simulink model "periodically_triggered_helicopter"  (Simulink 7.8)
settings: Solver=ode45  StartTime=0.0  StopTime=89  RelTol=1e-3
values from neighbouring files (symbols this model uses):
  d = lambda*0.5    [main_epsilon.m]    (also in main_rho_tau.m = 0.5)
undefined symbols (not defined in the file or in its folder): Ac_epsilon, Ac_rho, Ac_tau, c_epsilon, DiscIntNeverNeededParam, epsilon_0, Epsilon_disc, g, J_epsilon, Ka, Kb, Kc, L_epsilon, L_rho, L_tau, la, lh, lw, m, M, M_bf, Rho_disc, Tau_disc
libraries: simulink x6, commnoisgen2 x6, dspswit3 x3

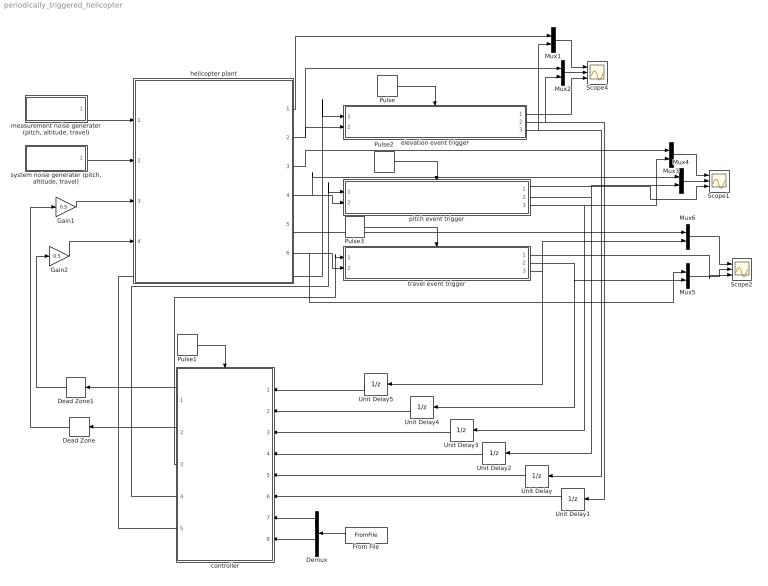
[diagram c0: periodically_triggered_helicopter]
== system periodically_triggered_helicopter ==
  Dead Zone : DeadZone  LowerValue=-1  UpperValue=1
  Dead Zone1 : DeadZone  LowerValue=-1  UpperValue=1
  Demux : Demux  Outputs=2
  From File : FromFile  FileName=input.mat  SampleTime=0
  Gain1 : Gain  Gain=0.5
  Gain2 : Gain  Gain=0.5
  Mux{1..6} (6 alike) : Mux  Inputs=2
  Pulse : DiscretePulseGenerator  PulseType=Time based  Period=0.005  PulseWidth=50
  Pulse1 : DiscretePulseGenerator  PulseType=Time based  Period=0.005  PulseWidth=30
  Pulse2 : DiscretePulseGenerator  PulseType=Time based  Period=0.005  PulseWidth=50
  Pulse3 : DiscretePulseGenerator  PulseType=Time based  Period=0.005  PulseWidth=50
  Scope1 : Scope  NumInputPorts=3
  Scope2 : Scope  NumInputPorts=3
  Scope4 : Scope  NumInputPorts=3
  Unit Delay{,1..5} (6 alike) : UnitDelay  SampleTime=-1
  controller : Subsystem
  elevation event trigger : Subsystem
  helicopter plant : Subsystem
  "measurement noise generater (pitch, altitude, travel)" : Subsystem
  pitch event trigger : Subsystem
  "system noise generater (pitch, altitude, travel)" : Subsystem
  travel event trigger : Subsystem
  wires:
  helicopter plant/2(altitude) -> elevation event trigger/2(elevation), Mux2/1
  Pulse/1 -> elevation event trigger/Trigger
  Mux1/1 -> Scope4/1
  Pulse1/1 -> controller/Trigger
  helicopter plant/5(travel rate) -> Mux6/1
  helicopter plant/3(pitch rate) -> Mux3/1
  controller/1(Vb) -> Dead Zone1/1
  Gain2/1 -> helicopter plant/4(Tb)
  controller/2(Vf) -> Dead Zone/1
  Gain1/1 -> helicopter plant/3(Tf)
  controller/5(u_elv) -> elevation event trigger/1(u_elv)
  From File/1 -> Demux/1
  Demux/2 -> controller/8(travel_rate_offset)
  Demux/1 -> controller/7(elevation_offset)
  helicopter plant/1(altitude rate) -> Mux1/1
  Mux2/1 -> Scope4/2
  elevation event trigger/3(remote estimated elevation rate) -> Unit Delay/1, Mux1/2
  elevation event trigger/2(remote estimated elevation) -> Unit Delay1/1, Mux2/2
  elevation event trigger/1(elevation transmission times) -> Scope4/3
  Pulse2/1 -> pitch event trigger/Trigger
  Unit Delay/1 -> controller/5(elevation_rate)
  Unit Delay1/1 -> controller/6(elevation)
  helicopter plant/4(pitch) -> pitch event trigger/2(pitch), Mux4/1
  pitch event trigger/2(remote estimated pitch) -> Unit Delay2/1, Mux4/2
  Unit Delay2/1 -> controller/4(pitch)
  pitch event trigger/3(remote estimated pitch rate) -> Mux3/2, Unit Delay3/1
  Mux3/1 -> Scope1/1
  Mux4/1 -> Scope1/2
  pitch event trigger/1(pitch transmission interval) -> Scope1/3
  Pulse3/1 -> travel event trigger/Trigger
  helicopter plant/6(travel) -> travel event trigger/2(travel), Mux5/1
  controller/3(u_trv) -> travel event trigger/1(u_trv)
  controller/4(u_pth) -> pitch event trigger/1(u_pth)
  Mux5/1 -> Scope2/2
  travel event trigger/2("remote estimated travel ") -> Unit Delay4/1, Mux5/2
  Unit Delay3/1 -> controller/3(pitch_rate)
  Unit Delay4/1 -> controller/2(travel)
  travel event trigger/3(remote estimated travel rate) -> Mux6/2, Unit Delay5/1
  Mux6/1 -> Scope2/1
  travel event trigger/1(travel transmission interval) -> Scope2/3
  Unit Delay5/1 -> controller/1(travel_rate)
  "measurement noise generater (pitch, altitude, travel)"/1(measurement noise) -> helicopter plant/1("measurement noise (pitch, altitude, travel)")
  "system noise generater (pitch, altitude, travel)"/1(system noise) -> helicopter plant/2("system noise (pitch, altitude, travel)")
  Dead Zone/1 -> Gain1/1
  Dead Zone1/1 -> Gain2/1

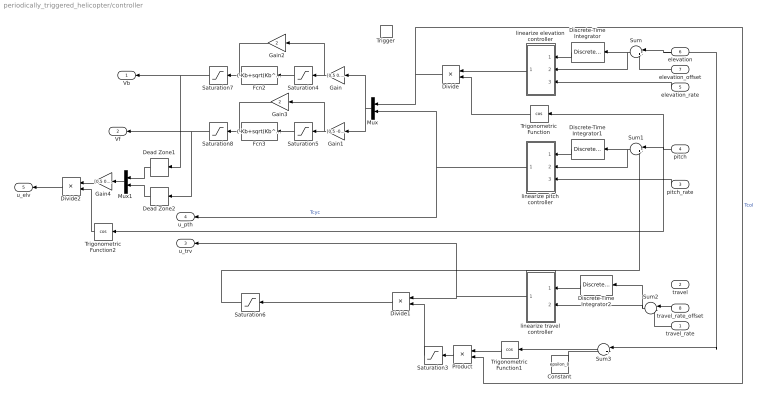
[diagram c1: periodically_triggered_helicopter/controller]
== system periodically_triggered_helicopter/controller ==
  travel_rate : Inport
  travel : Inport  Port=2
  pitch_rate : Inport  Port=3
  pitch : Inport  Port=4
  elevation_rate : Inport  Port=5
  elevation : Inport  Port=6
  elevation_offset : Inport  Port=7
  travel_rate_offset : Inport  Port=8
  Trigger : TriggerPort
  Constant : Constant  Value=epsilon_0
  Dead Zone1 : DeadZone  LowerValue=-1  UpperValue=1
  Dead Zone2 : DeadZone  LowerValue=-1  UpperValue=1
  Discrete-Time Integrator : DiscreteIntegrator  SampleTime=-1  LimitOutput=on  UpperSaturationLimit=1.8  LowerSaturationLimit=-1.8  ICPrevOutput=DiscIntNeverNeededParam  ICPrevScaledInput=DiscIntNeverNeededParam
  Discrete-Time Integrator1 : DiscreteIntegrator  SampleTime=-1  LimitOutput=on  UpperSaturationLimit=0.5  LowerSaturationLimit=-0.5  ICPrevOutput=DiscIntNeverNeededParam  ICPrevScaledInput=DiscIntNeverNeededParam
  Discrete-Time Integrator2 : DiscreteIntegrator  SampleTime=-1  LimitOutput=on  UpperSaturationLimit=0.12  LowerSaturationLimit=-0.12  ICPrevOutput=DiscIntNeverNeededParam  ICPrevScaledInput=DiscIntNeverNeededParam
  Divide : Product  Inputs=*/
  Divide1 : Product  Inputs=*/
  Divide2 : Product  Inputs=**
  Fcn2 : Fcn  Expr=(-Kb+sqrt(Kb^2-4*Ka*(Kc-u(1))))/(2*Ka)
  Fcn3 : Fcn  Expr=(-Kb+sqrt(Kb^2-4*Ka*(Kc-u(1))))/(2*Ka)
  Gain : Gain  Gain=[0.5 0.5]  Multiplication=Matrix(K*u)
  Gain1 : Gain  Gain=[0.5 -0.5]  Multiplication=Matrix(K*u)
  Gain2 : Gain  Gain=2
  Gain3 : Gain  Gain=2
  Gain4 : Gain  Gain=[0.5 0.5]  Multiplication=Matrix(K*u)
  Mux : Mux  Inputs=2
  Mux1 : Mux  Inputs=2
  Product : Product
  Saturation3 : Saturate  UpperLimit=inf  LowerLimit=0.8
  Saturation4 : Saturate  UpperLimit=1  LowerLimit=-0.0012
  Saturation5 : Saturate  UpperLimit=1  LowerLimit=-0.0012
  Saturation6 : Saturate  UpperLimit=0.6  LowerLimit=-0.6
  Saturation7 : Saturate  UpperLimit=4.99  LowerLimit=-4.99
  Saturation8 : Saturate  UpperLimit=4.99  LowerLimit=-4.99
  Sum : Sum  Inputs=|+-
  Sum1 : Sum  Inputs=|+-
  Sum2 : Sum  Inputs=|-+
  Sum3 : Sum  Inputs=|+-
  Trigonometric Function : Trigonometry  Operator=cos
  Trigonometric Function1 : Trigonometry  Operator=cos
  Trigonometric Function2 : Trigonometry  Operator=cos
  linearize elevation controller : Subsystem
  linearize pitch controller : Subsystem
  linearize travel controller : Subsystem
  Vb : Outport
  Vf : Outport  Port=2
  u_trv : Outport  Port=3
  u_pth : Outport  Port=4
  u_elv : Outport  Port=5
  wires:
  elevation/1 -> Sum/1, Sum3/1
  elevation_offset/1 -> Sum/2
  Sum/1 -> linearize elevation controller/2(P), Discrete-Time Integrator/1
  Discrete-Time Integrator/1 -> linearize elevation controller/1(I)
  elevation_rate/1 -> linearize elevation controller/3(D)
  pitch/1 -> Sum1/1, Trigonometric Function/1, Trigonometric Function2/1
  Sum1/1 -> linearize pitch controller/2(P), Discrete-Time Integrator1/1
  pitch_rate/1 -> linearize pitch controller/3(D)
  travel_rate_offset/1 -> Sum2/1
  travel_rate/1 -> Sum2/2
  Sum2/1 -> Discrete-Time Integrator2/1, linearize travel controller/2(P)
  Discrete-Time Integrator2/1 -> linearize travel controller/1(I)
  Sum3/1 -> Trigonometric Function1/1
  Trigonometric Function1/1 -> Product/1
  Divide/1 -> Mux/1, Product/2  "Tcol"
  Product/1 -> Saturation3/1
  Saturation3/1 -> Divide1/2
  Mux/1 -> Gain/1, Gain1/1
  Gain/1 -> Saturation4/1, Gain2/1
  Gain1/1 -> Saturation5/1, Gain3/1
  Divide1/1 -> Saturation6/1
  Saturation6/1 -> Sum1/2
  Saturation7/1 -> Vb/1, Dead Zone1/1
  Saturation8/1 -> Vf/1, Dead Zone2/1
  Constant/1 -> Sum3/2
  Saturation4/1 -> Fcn2/1
  Saturation5/1 -> Fcn3/1
  Trigonometric Function/1 -> Divide/2
  Discrete-Time Integrator1/1 -> linearize pitch controller/1(I)
  Gain2/1 -> Saturation7/1
  Gain3/1 -> Saturation8/1
  linearize pitch controller/1(u_pth) -> Mux/2, u_pth/1  "Tcyc"
  linearize travel controller/1(u_trv) -> Divide1/1, u_trv/1
  linearize elevation controller/1(u_elv) -> Divide/1
  Dead Zone1/1 -> Mux1/1
  Dead Zone2/1 -> Mux1/2
  Mux1/1 -> Gain4/1
  Gain4/1 -> Divide2/1
  Trigonometric Function2/1 -> Divide2/2
  Divide2/1 -> u_elv/1

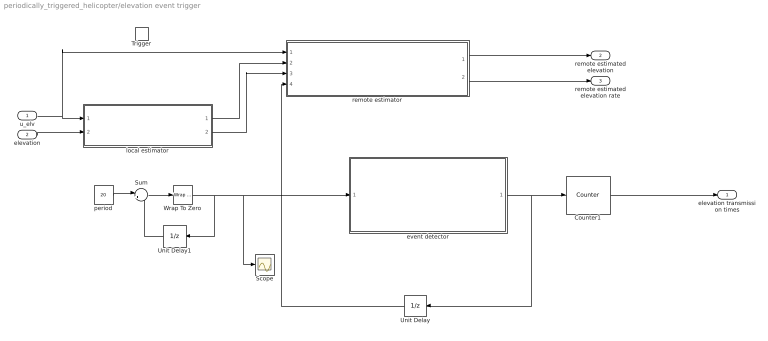
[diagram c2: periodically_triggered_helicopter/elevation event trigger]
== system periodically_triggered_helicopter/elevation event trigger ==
  u_elv : Inport
  elevation : Inport  Port=2
  Trigger : TriggerPort
  Counter1 : dspswit3/Counter  Direction=Up  CountEvent=Non-zero sample  CounterSize=User defined  MaxCount=20000  InitialCount=0  Output=Count  HitValue=32  ResetInput=off  SamplesPerFrame=1  Ts=1  CntDtype=int32  HitDtype=Logical
  Scope : Scope
  Sum : Sum  Inputs=|++
  Unit Delay : UnitDelay  SampleTime=-1
  Unit Delay1 : UnitDelay  SampleTime=-1
  Wrap To Zero : simulink/Discontinuities/Wrap To Zero  Threshold=4
  event detector : Subsystem
  local estimator : Subsystem
  period : Constant  Value=20
  remote estimator : Subsystem
  elevation transmission times : Outport
  remote estimated elevation : Outport  Port=2
  remote estimated elevation rate : Outport  Port=3
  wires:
  u_elv/1 -> local estimator/1(u_elv), remote estimator/1(u_elv)
  elevation/1 -> local estimator/2(elevation)
  local estimator/1(local estimated elevation) -> remote estimator/2("local estimated elevation ")
  remote estimator/1(remote estimated elevation) -> remote estimated elevation/1
  local estimator/2(local estimated elevation rate) -> remote estimator/3(local estimated elevation rate)
  event detector/1(transmit signal) -> Unit Delay/1, Counter1/1
  Counter1/1 -> elevation transmission times/1
  Unit Delay/1 -> remote estimator/4(transmit signal)
  remote estimator/2(remote estimated elevation rate) -> remote estimated elevation rate/1
  period/1 -> Sum/1
  Sum/1 -> Wrap To Zero/1
  Wrap To Zero/1 -> event detector/1(steps), Scope/1, Unit Delay1/1
  Unit Delay1/1 -> Sum/2

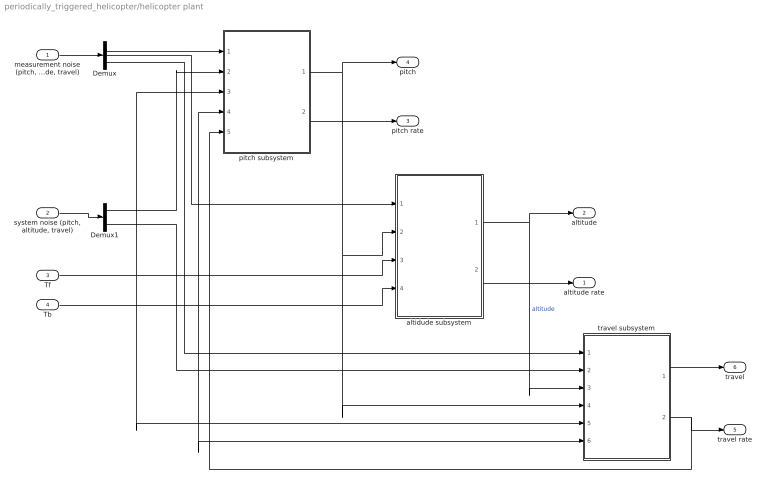
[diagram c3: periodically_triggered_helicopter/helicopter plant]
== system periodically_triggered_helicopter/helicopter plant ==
  "measurement noise (pitch, altitude, travel)" : Inport
  "system noise (pitch, altitude, travel)" : Inport  Port=2
  Tf : Inport  Port=3
  Tb : Inport  Port=4
  Demux : Demux  Outputs=3
  Demux1 : Demux  Outputs=3
  altidude subsystem : Subsystem
  pitch subsystem : Subsystem
  travel subsystem : Subsystem
  altitude rate : Outport
  altitude : Outport  Port=2
  pitch rate : Outport  Port=3
  pitch : Outport  Port=4
  travel rate : Outport  Port=5
  travel : Outport  Port=6
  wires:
  pitch subsystem/1(pitch) -> pitch/1, altidude subsystem/2(pitch), travel subsystem/4(pitch)
  altidude subsystem/1(altitude) -> altitude/1, travel subsystem/3(altitude)  "altitude"
  pitch subsystem/2(pitch rate) -> pitch rate/1
  altidude subsystem/2(altitude rate) -> altitude rate/1
  travel subsystem/1(travel) -> travel/1
  travel subsystem/2(travel rate) -> pitch subsystem/5(travel_rate), travel rate/1
  Demux/1 -> pitch subsystem/1(measurement noise)
  Demux/2 -> altidude subsystem/1(measurement noise)
  Demux/3 -> travel subsystem/1(measurement noise)
  "measurement noise (pitch, altitude, travel)"/1 -> Demux/1
  Demux1/1 -> pitch subsystem/2(system noise)
  Demux1/3 -> travel subsystem/2(system noise)
  Tf/1 -> altidude subsystem/3(Tf), travel subsystem/5(Tf), pitch subsystem/3(Tf)
  Tb/1 -> altidude subsystem/4(Tb), pitch subsystem/4(Tb), travel subsystem/6(Tb)
  "system noise (pitch, altitude, travel)"/1 -> Demux1/1

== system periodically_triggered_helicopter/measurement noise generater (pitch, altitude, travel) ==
  Mux : Mux  Inputs=3
  altitude Noise Generator : commnoisgen2/Gaussian Noise Generator  m=0  d=1.857e-8  s=41  Ts=0.0025  frameBased=off  sampPerFrame=1  orient=off  outDataType=double
  pitch noise Generator : commnoisgen2/Gaussian Noise Generator  m=0  d=1.857e-8  s=1  Ts=0.0025  frameBased=off  sampPerFrame=1  orient=off  outDataType=double
  travel noise Generator : commnoisgen2/Gaussian Noise Generator  m=0  d=1.857e-8  s=3  Ts=0.0025  frameBased=off  sampPerFrame=1  orient=off  outDataType=double
  measurement noise : Outport
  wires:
  pitch noise Generator/1 -> Mux/1
  altitude Noise Generator/1 -> Mux/2
  travel noise Generator/1 -> Mux/3
  Mux/1 -> measurement noise/1

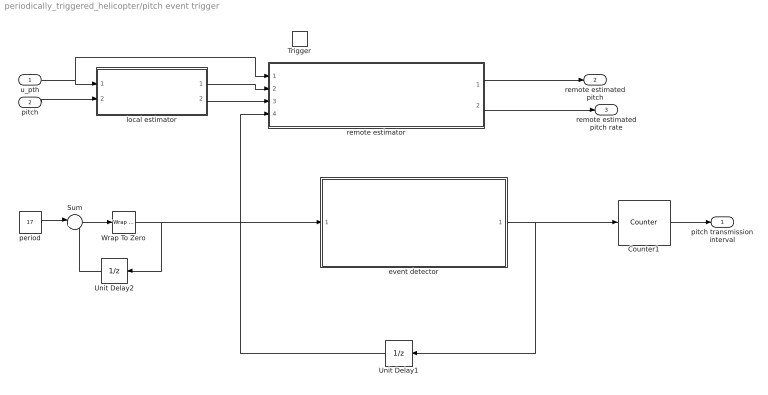
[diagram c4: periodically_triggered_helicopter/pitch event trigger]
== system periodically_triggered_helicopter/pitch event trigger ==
  u_pth : Inport
  pitch : Inport  Port=2
  Trigger : TriggerPort
  Counter1 : dspswit3/Counter  Direction=Up  CountEvent=Non-zero sample  CounterSize=User defined  MaxCount=20000  InitialCount=0  Output=Count  HitValue=32  ResetInput=off  SamplesPerFrame=1  Ts=1  CntDtype=int32  HitDtype=Logical
  Sum : Sum  Inputs=|++
  Unit Delay1 : UnitDelay  SampleTime=-1
  Unit Delay2 : UnitDelay  SampleTime=-1
  Wrap To Zero : simulink/Discontinuities/Wrap To Zero  Threshold=1
  event detector : Subsystem
  local estimator : Subsystem
  period : Constant  Value=17
  remote estimator : Subsystem
  pitch transmission interval : Outport
  remote estimated pitch : Outport  Port=2
  remote estimated pitch rate : Outport  Port=3
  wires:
  u_pth/1 -> local estimator/1(u_pth), remote estimator/1(u_pth)
  pitch/1 -> local estimator/2(pitch)
  local estimator/1(local estimated pitch) -> remote estimator/2(local estimated pitch)
  local estimator/2(local estimated pitch rate) -> remote estimator/3(local estimated pitch rate)
  remote estimator/1(remote estimated elevation) -> remote estimated pitch/1
  remote estimator/2(remote estimated elevation rate) -> remote estimated pitch rate/1
  Counter1/1 -> pitch transmission interval/1
  event detector/1(transmit signal) -> Unit Delay1/1, Counter1/1
  Unit Delay1/1 -> remote estimator/4(transmit signal)
  period/1 -> Sum/1
  Sum/1 -> Wrap To Zero/1
  Wrap To Zero/1 -> Unit Delay2/1, event detector/1(steps)
  Unit Delay2/1 -> Sum/2

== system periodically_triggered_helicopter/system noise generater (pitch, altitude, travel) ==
  Mux : Mux  Inputs=3
  altitude Noise Generator : commnoisgen2/Gaussian Noise Generator  m=0  d=1e-12  s=7  Ts=0.0025  frameBased=off  sampPerFrame=1  orient=off  outDataType=double
  pitch noise Generator : commnoisgen2/Gaussian Noise Generator  m=0  d=1e-12  s=5  Ts=0.0025  frameBased=off  sampPerFrame=1  orient=off  outDataType=double
  travel Noise Generator : commnoisgen2/Gaussian Noise Generator  m=0  d=1e-12  s=11  Ts=0.0025  frameBased=off  sampPerFrame=1  orient=off  outDataType=double
  system noise : Outport
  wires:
  pitch noise Generator/1 -> Mux/1
  altitude Noise Generator/1 -> Mux/2
  Mux/1 -> system noise/1
  travel Noise Generator/1 -> Mux/3

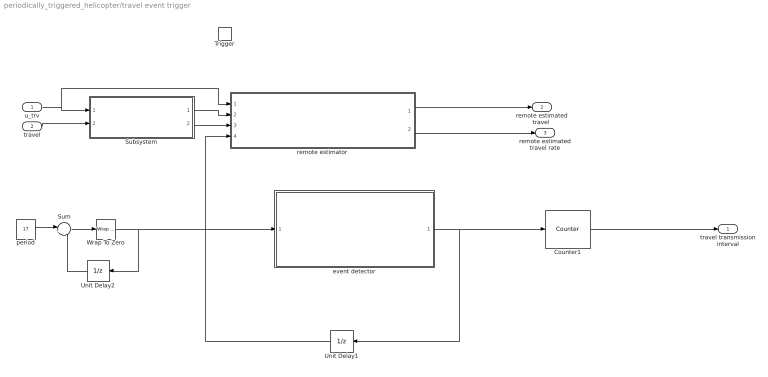
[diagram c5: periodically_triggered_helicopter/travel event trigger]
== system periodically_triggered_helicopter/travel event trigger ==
  u_trv : Inport
  travel : Inport  Port=2
  Trigger : TriggerPort
  Counter1 : dspswit3/Counter  Direction=Up  CountEvent=Non-zero sample  CounterSize=User defined  MaxCount=20000  InitialCount=0  Output=Count  HitValue=32  ResetInput=off  SamplesPerFrame=1  Ts=1  CntDtype=int32  HitDtype=Logical
  Subsystem : Subsystem
  Sum : Sum  Inputs=|++
  Unit Delay1 : UnitDelay  SampleTime=-1
  Unit Delay2 : UnitDelay  SampleTime=-1
  Wrap To Zero : simulink/Discontinuities/Wrap To Zero  Threshold=2
  event detector : Subsystem
  period : Constant  Value=17
  remote estimator : Subsystem
  travel transmission interval : Outport
  "remote estimated travel " : Outport  Port=2
  remote estimated travel rate : Outport  Port=3
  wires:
  u_trv/1 -> Subsystem/1(u_trv), remote estimator/1(u_trv)
  travel/1 -> Subsystem/2(travel)
  Subsystem/2(local estimated travel rate) -> remote estimator/3(local estimated travel rate)
  remote estimator/2(remote estimated travel rate) -> remote estimated travel rate/1
  remote estimator/1(remote estimated travel) -> "remote estimated travel "/1
  Subsystem/1(local estimated travel) -> remote estimator/2(local estimated travel)
  Counter1/1 -> travel transmission interval/1
  event detector/1(transmit signal) -> Unit Delay1/1, Counter1/1
  Unit Delay1/1 -> remote estimator/4(transmit signal)
  period/1 -> Sum/1
  Sum/1 -> Wrap To Zero/1
  Wrap To Zero/1 -> Unit Delay2/1, event detector/1(steps)
  Unit Delay2/1 -> Sum/2

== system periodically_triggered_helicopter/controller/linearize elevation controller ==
  I : Inport
  P : Inport  Port=2
  D : Inport  Port=3
  Gain : Gain  Gain=[-7 -44 -68]  Multiplication=Matrix(K*u)
  Mux : Mux  Inputs=3
  u_elv : Outport
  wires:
  Mux/1 -> Gain/1
  I/1 -> Mux/1
  Gain/1 -> u_elv/1
  P/1 -> Mux/2
  D/1 -> Mux/3

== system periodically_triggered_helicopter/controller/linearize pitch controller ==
  I : Inport
  P : Inport  Port=2
  D : Inport  Port=3
  Gain : Gain  Gain=[-3.5 -30 -20]  Multiplication=Matrix(K*u)
  Mux : Mux  Inputs=3
  u_pth : Outport
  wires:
  Mux/1 -> Gain/1
  I/1 -> Mux/1
  Gain/1 -> u_pth/1
  P/1 -> Mux/2
  D/1 -> Mux/3

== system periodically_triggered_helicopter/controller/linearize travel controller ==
  I : Inport
  P : Inport  Port=2
  Gain : Gain  Gain=[5 30]  Multiplication=Matrix(K*u)
  Mux : Mux  Inputs=2
  u_trv : Outport
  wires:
  Mux/1 -> Gain/1
  I/1 -> Mux/1
  Gain/1 -> u_trv/1
  P/1 -> Mux/2

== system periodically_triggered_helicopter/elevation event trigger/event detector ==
  steps : Inport
  Compare To Constant : simulink/Logic and Bit Operations/Compare To Constant  relop===  const=0  OutDataTypeStr=uint8
  transmit signal : Outport
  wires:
  steps/1 -> Compare To Constant/1
  Compare To Constant/1 -> transmit signal/1

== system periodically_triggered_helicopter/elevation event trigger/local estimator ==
  u_elv : Inport
  elevation : Inport  Port=2
  Demux : Demux  Outputs=2
  Gain2 : Gain  Gain=[Ac_epsilon(2:3,2:3) Epsilon_disc.B(2:3) L_epsilon(2:3,2)]  Multiplication=Matrix(K*u)
  Mux : Mux  Inputs=3
  Unit Delay : UnitDelay  SampleTime=-1
  local estimated elevation : Outport
  local estimated elevation rate : Outport  Port=2
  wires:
  Unit Delay/1 -> Mux/1
  u_elv/1 -> Mux/2
  elevation/1 -> Mux/3
  Mux/1 -> Gain2/1
  Gain2/1 -> Demux/1, Unit Delay/1
  Demux/1 -> local estimated elevation/1
  Demux/2 -> local estimated elevation rate/1

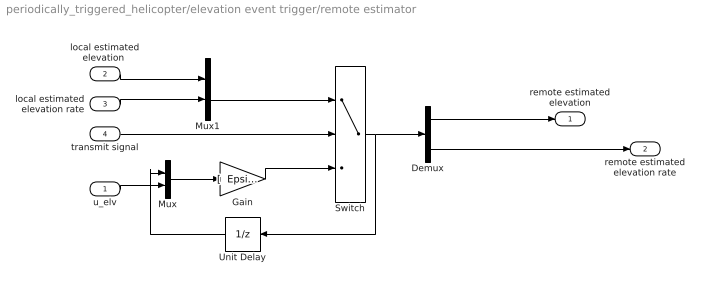
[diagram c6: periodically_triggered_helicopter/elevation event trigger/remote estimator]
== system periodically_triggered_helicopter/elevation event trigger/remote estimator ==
  u_elv : Inport
  "local estimated elevation " : Inport  Port=2
  local estimated elevation rate : Inport  Port=3
  transmit signal : Inport  Port=4
  Demux : Demux  Outputs=2
  Gain : Gain  Gain="[  Epsilon_disc.A(2:3,2:3)  Epsilon_disc.B(2:3)]"  Multiplication=Matrix(K*u)
  Mux : Mux  Inputs=2
  Mux1 : Mux  Inputs=2
  Switch : Switch  Threshold=1
  Unit Delay : UnitDelay  SampleTime=-1
  remote estimated elevation : Outport
  remote estimated elevation rate : Outport  Port=2
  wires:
  Mux/1 -> Gain/1
  u_elv/1 -> Mux/2
  Demux/1 -> remote estimated elevation/1
  Demux/2 -> remote estimated elevation rate/1
  Gain/1 -> Switch/3
  transmit signal/1 -> Switch/2
  Switch/1 -> Demux/1, Unit Delay/1
  Unit Delay/1 -> Mux/1
  "local estimated elevation "/1 -> Mux1/1
  local estimated elevation rate/1 -> Mux1/2
  Mux1/1 -> Switch/1

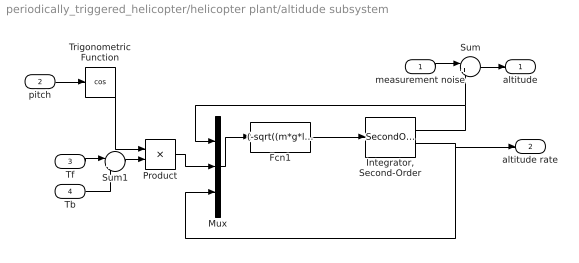
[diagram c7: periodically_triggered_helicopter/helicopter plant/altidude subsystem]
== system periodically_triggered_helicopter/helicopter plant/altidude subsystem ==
  measurement noise : Inport
  pitch : Inport  Port=2
  Tf : Inport  Port=3
  Tb : Inport  Port=4
  Fcn1 : Fcn  Expr=(-sqrt((m*g*lw-M*g*la)^2+((m+M)*g*d)^2)*sin(u(1))+(la+d*tan(u(1)+epsilon_0))*u(2)-c_epsilon*u(3))/J_epsilon
  "Integrator, Second-Order" : SecondOrderIntegrator
  Mux : Mux  Inputs=3
  Product : Product
  Sum : Sum  Inputs=|++
  Sum1 : Sum  Inputs=|++
  Trigonometric Function : Trigonometry  Operator=cos
  altitude : Outport
  altitude rate : Outport  Port=2
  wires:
  Fcn1/1 -> "Integrator, Second-Order"/1
  "Integrator, Second-Order"/1 -> Sum/2, Mux/1
  measurement noise/1 -> Sum/1
  Sum/1 -> altitude/1
  "Integrator, Second-Order"/2 -> altitude rate/1, Mux/3
  Tf/1 -> Sum1/1
  Tb/1 -> Sum1/2
  Mux/1 -> Fcn1/1
  Sum1/1 -> Product/2
  pitch/1 -> Trigonometric Function/1
  Product/1 -> Mux/2
  Trigonometric Function/1 -> Product/1

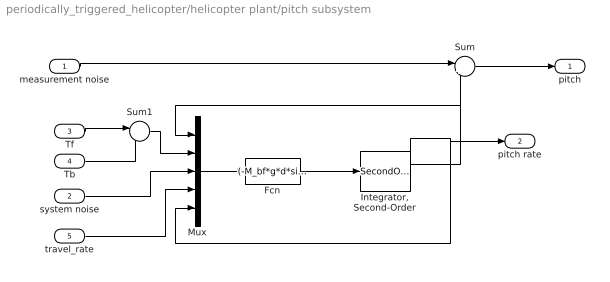
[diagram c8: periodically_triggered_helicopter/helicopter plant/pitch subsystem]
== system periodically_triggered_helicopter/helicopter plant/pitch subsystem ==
  measurement noise : Inport
  system noise : Inport  Port=2
  Tf : Inport  Port=3
  Tb : Inport  Port=4
  travel_rate : Inport  Port=5
  Fcn : Fcn  Expr=(-M_bf*g*d*sin(u(1))+lh*u(2)-0.003*u(5)+0.003*u(4)+u(3))/(0.01)
  "Integrator, Second-Order" : SecondOrderIntegrator
  Mux : Mux  Inputs=5
  Sum : Sum  Inputs=|++
  Sum1 : Sum  Inputs=|-+
  pitch : Outport
  pitch rate : Outport  Port=2
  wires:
  Mux/1 -> Fcn/1
  Fcn/1 -> "Integrator, Second-Order"/1
  "Integrator, Second-Order"/1 -> Sum/2, Mux/1
  measurement noise/1 -> Sum/1
  Sum/1 -> pitch/1
  "Integrator, Second-Order"/2 -> pitch rate/1, Mux/5
  system noise/1 -> Mux/3
  Tf/1 -> Sum1/1
  Tb/1 -> Sum1/2
  travel_rate/1 -> Mux/4
  Sum1/1 -> Mux/2

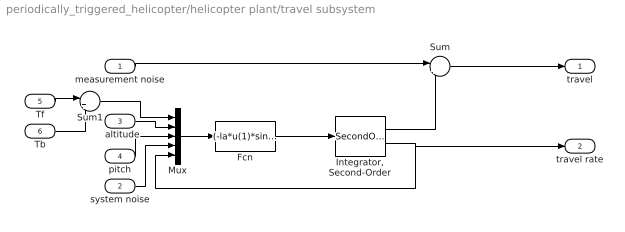
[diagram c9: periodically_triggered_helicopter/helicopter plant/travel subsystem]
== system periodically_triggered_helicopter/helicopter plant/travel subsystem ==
  measurement noise : Inport
  system noise : Inport  Port=2
  altitude : Inport  Port=3
  pitch : Inport  Port=4
  Tf : Inport  Port=5
  Tb : Inport  Port=6
  Fcn : Fcn  Expr=(-la*u(1)*sin(u(3))*cos(u(2)+epsilon_0)-0.25*u(5)+u(4))/4
  "Integrator, Second-Order" : SecondOrderIntegrator
  Mux : Mux  Inputs=5
  Sum : Sum  Inputs=|++
  Sum1 : Sum  Inputs=|++
  travel : Outport
  travel rate : Outport  Port=2
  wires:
  Mux/1 -> Fcn/1
  "Integrator, Second-Order"/1 -> Sum/2
  measurement noise/1 -> Sum/1
  Sum/1 -> travel/1
  altitude/1 -> Mux/2
  "Integrator, Second-Order"/2 -> travel rate/1, Mux/5
  Sum1/1 -> Mux/1
  pitch/1 -> Mux/3
  system noise/1 -> Mux/4
  Tf/1 -> Sum1/1
  Tb/1 -> Sum1/2
  Fcn/1 -> "Integrator, Second-Order"/1

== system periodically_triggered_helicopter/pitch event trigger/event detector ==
  steps : Inport
  Compare To Constant : simulink/Logic and Bit Operations/Compare To Constant  relop===  const=0  OutDataTypeStr=uint8
  transmit signal : Outport
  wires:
  steps/1 -> Compare To Constant/1
  Compare To Constant/1 -> transmit signal/1

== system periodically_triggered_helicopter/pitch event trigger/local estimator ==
  u_pth : Inport
  pitch : Inport  Port=2
  Demux : Demux  Outputs=2
  Gain2 : Gain  Gain=[Ac_rho(2:3,2:3) Rho_disc.B(2:3) L_rho(2:3,2)]  Multiplication=Matrix(K*u)
  Mux : Mux  Inputs=3
  Unit Delay : UnitDelay  SampleTime=-1
  local estimated pitch : Outport
  local estimated pitch rate : Outport  Port=2
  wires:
  Gain2/1 -> Unit Delay/1, Demux/1
  Unit Delay/1 -> Mux/1
  Mux/1 -> Gain2/1
  u_pth/1 -> Mux/2
  pitch/1 -> Mux/3
  Demux/1 -> local estimated pitch/1
  Demux/2 -> local estimated pitch rate/1

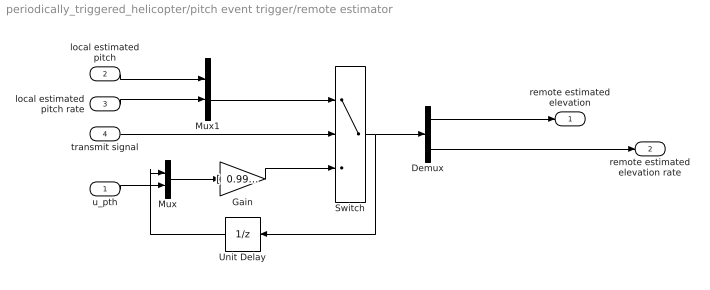
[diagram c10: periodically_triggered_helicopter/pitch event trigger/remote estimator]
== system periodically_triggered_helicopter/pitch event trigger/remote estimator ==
  u_pth : Inport
  local estimated pitch : Inport  Port=2
  local estimated pitch rate : Inport  Port=3
  transmit signal : Inport  Port=4
  Demux : Demux  Outputs=2
  Gain : Gain  Gain=|  Multiplication=Matrix(K*u)
      | [  0.9999    0.0050    0.0002
      | ;   -0.0568    0.9984    0.0884]
  Mux : Mux  Inputs=2
  Mux1 : Mux  Inputs=2
  Switch : Switch  Threshold=0.8
  Unit Delay : UnitDelay  SampleTime=-1
  remote estimated elevation : Outport
  remote estimated elevation rate : Outport  Port=2
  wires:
  Mux/1 -> Gain/1
  u_pth/1 -> Mux/2
  Demux/1 -> remote estimated elevation/1
  Demux/2 -> remote estimated elevation rate/1
  Gain/1 -> Switch/3
  transmit signal/1 -> Switch/2
  Switch/1 -> Unit Delay/1, Demux/1
  Unit Delay/1 -> Mux/1
  local estimated pitch/1 -> Mux1/1
  local estimated pitch rate/1 -> Mux1/2
  Mux1/1 -> Switch/1

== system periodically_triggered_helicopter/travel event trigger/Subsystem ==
  u_trv : Inport
  travel : Inport  Port=2
  Demux : Demux  Outputs=2
  Gain2 : Gain  Gain=[Ac_tau Tau_disc.B L_tau]  Multiplication=Matrix(K*u)
  Mux : Mux  Inputs=3
  Unit Delay : UnitDelay  SampleTime=-1
  local estimated travel : Outport
  local estimated travel rate : Outport  Port=2
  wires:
  Gain2/1 -> Unit Delay/1, Demux/1
  Unit Delay/1 -> Mux/1
  Mux/1 -> Gain2/1
  u_trv/1 -> Mux/2
  travel/1 -> Mux/3
  Demux/1 -> local estimated travel/1
  Demux/2 -> local estimated travel rate/1

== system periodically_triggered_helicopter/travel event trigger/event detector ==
  steps : Inport
  Compare To Constant : simulink/Logic and Bit Operations/Compare To Constant  relop===  const=0  OutDataTypeStr=uint8
  transmit signal : Outport
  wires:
  steps/1 -> Compare To Constant/1
  Compare To Constant/1 -> transmit signal/1

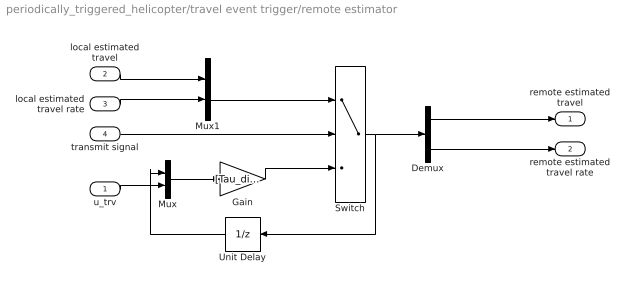
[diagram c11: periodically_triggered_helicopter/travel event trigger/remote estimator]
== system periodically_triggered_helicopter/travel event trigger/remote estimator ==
  u_trv : Inport
  local estimated travel : Inport  Port=2
  local estimated travel rate : Inport  Port=3
  transmit signal : Inport  Port=4
  Demux : Demux  Outputs=2
  Gain : Gain  Gain=[Tau_disc.A Tau_disc.B]  Multiplication=Matrix(K*u)
  Mux : Mux  Inputs=2
  Mux1 : Mux  Inputs=2
  Switch : Switch  Threshold=0.8
  Unit Delay : UnitDelay  SampleTime=-1
  remote estimated travel : Outport
  remote estimated travel rate : Outport  Port=2
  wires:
  Mux/1 -> Gain/1
  u_trv/1 -> Mux/2
  Demux/1 -> remote estimated travel/1
  Demux/2 -> remote estimated travel rate/1
  Gain/1 -> Switch/3
  transmit signal/1 -> Switch/2
  Switch/1 -> Unit Delay/1, Demux/1
  Unit Delay/1 -> Mux/1
  local estimated travel/1 -> Mux1/1
  local estimated travel rate/1 -> Mux1/2
  Mux1/1 -> Switch/1
